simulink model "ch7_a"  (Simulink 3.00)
settings: Solver=ode23  SolverMode=SingleTasking  StartTime=0.0  StopTime=1000  MaxStep=10  RelTol=1e-3  AbsTol=1e-6
libraries: simulink3 x1

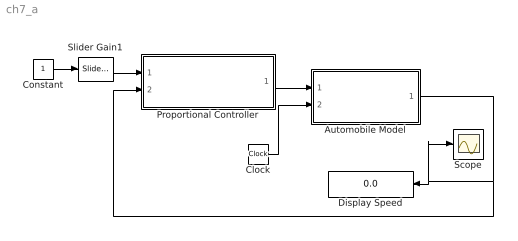
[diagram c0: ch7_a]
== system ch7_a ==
  Automobile Model : Subsystem
  Clock : Clock
  Constant : Constant  Value=1
  Display Speed : Display
  Proportional Controller : Subsystem
  Scope : Scope
  Slider Gain1 : simulink3/Math/Slider Gain  low=0  gain=70  high=100
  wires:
  Automobile Model/1(Speed Out) -> Scope/1, Display Speed/1, Proportional Controller/2(Actual Speed)
  Proportional Controller/1(Commanded Thrust) -> Automobile Model/1(Commanded Thrust)
  Constant/1 -> Slider Gain1/1
  Clock/1 -> Automobile Model/2(Time In)
  Slider Gain1/1 -> Proportional Controller/1(Desired Speed)

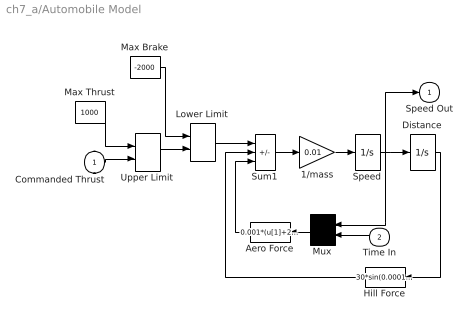
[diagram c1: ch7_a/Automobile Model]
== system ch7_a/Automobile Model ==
  Commanded Thrust : Inport  Port=1  PortWidth=-1  SampleTime=-1  DataType=auto
  Time In : Inport  Orientation=left  Port=2  PortWidth=-1  SampleTime=-1  DataType=auto
  1/mass : Gain  Gain=0.01  SaturateOnIntegerOverflow=on
  Aero Force : Fcn  Orientation=left  Expr=0.001*(u[1]+20*sin(0.01*u[2]))^2
  Distance : Integrator  ExternalReset=none  InitialConditionSource=internal  InitialCondition=0  LimitOutput=off  UpperSaturationLimit=inf  LowerSaturationLimit=-inf  ShowSaturationPort=off  ShowStatePort=off  AbsoluteTolerance=auto
  Hill Force : Fcn  Orientation=left  Expr=30*sin(0.0001*u[1])
  Lower Limit : MinMax  Function=max  Inputs=2
  Max Brake : Constant  Value=-2000
  Max Thrust : Constant  Value=1000
  Mux : Mux  Orientation=left  Inputs=2
  Speed : Integrator  ExternalReset=none  InitialConditionSource=internal  InitialCondition=0  LimitOutput=off  UpperSaturationLimit=inf  LowerSaturationLimit=-inf  ShowSaturationPort=off  ShowStatePort=off  AbsoluteTolerance=auto
  Sum1 : Sum  Inputs=+--  SaturateOnIntegerOverflow=on
  Upper Limit : MinMax  Function=min  Inputs=2
  Speed Out : Outport  Port=1  InitialOutput=0
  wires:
  Time In/1 -> Mux/2
  Lower Limit/1 -> Sum1/1
  Max Brake/1 -> Lower Limit/1
  Max Thrust/1 -> Upper Limit/1
  Upper Limit/1 -> Lower Limit/2
  1/mass/1 -> Speed/1
  Sum1/1 -> 1/mass/1
  Distance/1 -> Hill Force/1
  Hill Force/1 -> Sum1/2
  Aero Force/1 -> Sum1/3
  Speed/1 -> Mux/1, Speed Out/1, Distance/1
  Mux/1 -> Aero Force/1
  Commanded Thrust/1 -> Upper Limit/2

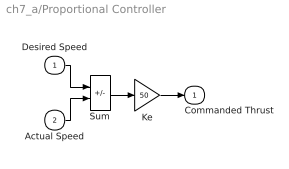
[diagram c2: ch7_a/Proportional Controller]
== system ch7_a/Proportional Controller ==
  Desired Speed : Inport  Port=1  PortWidth=-1  SampleTime=-1  DataType=auto
  Actual Speed : Inport  Port=2  PortWidth=-1  SampleTime=-1  DataType=auto
  Ke : Gain  Gain=50  SaturateOnIntegerOverflow=on
  Sum : Sum  Inputs=+-  SaturateOnIntegerOverflow=on
  Commanded Thrust : Outport  Port=1  InitialOutput=0
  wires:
  Actual Speed/1 -> Sum/2
  Sum/1 -> Ke/1
  Desired Speed/1 -> Sum/1
  Ke/1 -> Commanded Thrust/1
